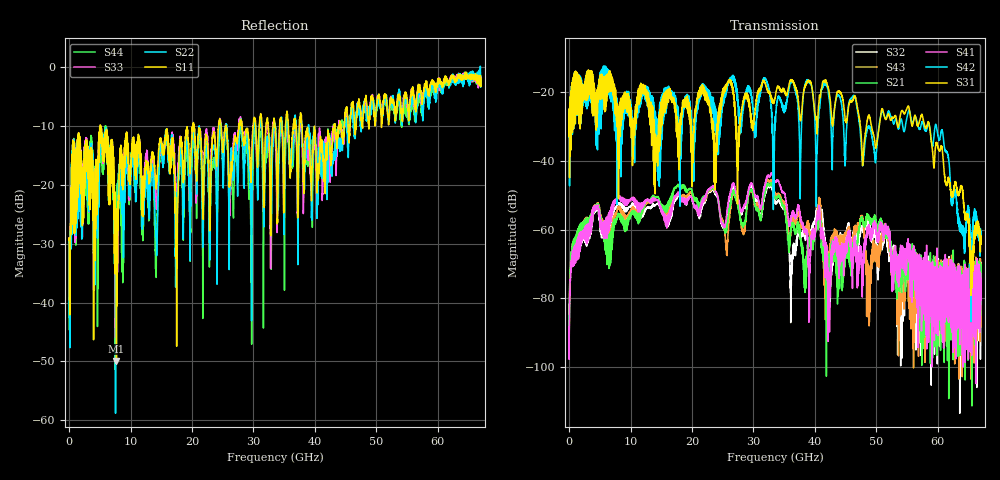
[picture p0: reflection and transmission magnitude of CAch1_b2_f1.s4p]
!Agilent Technologies,N5247A,US51170199,A.09.90.13
!Agilent N5247A: A.09.90.13
!Date: Thursday, October 18, 2018 12:09:48
!Correction: S11(Full 4 Port(1,2,3,4))
!S12(Full 4 Port(1,2,3,4))
!S13(Full 4 Port(1,2,3,4))
!S14(Full 4 Port(1,2,3,4))
!S21(Full 4 Port(1,2,3,4))
!S22(Full 4 Port(1,2,3,4))
!S23(Full 4 Port(1,2,3,4))
!S24(Full 4 Port(1,2,3,4))
!S31(Full 4 Port(1,2,3,4))
!S32(Full 4 Port(1,2,3,4))
!S33(Full 4 Port(1,2,3,4))
!S34(Full 4 Port(1,2,3,4))
!S41(Full 4 Port(1,2,3,4))
!S42(Full 4 Port(1,2,3,4))
!S43(Full 4 Port(1,2,3,4))
!S44(Full 4 Port(1,2,3,4))
!S4P File: Measurements: <S11,S12,S13,S14>,
!<S21,S22,S23,S24>,
!<S31,S32,S33,S34>,
!<S41,S42,S43,S44>:
# Hz S  dB  R 50
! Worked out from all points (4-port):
!   6701 points, 10 MHz to 67 GHz, reference 50 ohm
!   strongest paths, dB at 10 MHz, 16.76 GHz, 33.51 GHz, 50.25 GHz, 67 GHz:
!     S31: -32.9, -22.8, -21.9, -32.7, -63.0
!     S42: -33.1, -20.0, -29.9, -32.3, -62.8
!     S41: -88.2, -54.2, -46.0, -61.6, -80.5
!     S21: -87.9, -50.6, -50.5, -60.2, -77.4
!     S43: -87.8, -53.1, -49.3, -66.8, -77.2
!     S32: -81.7, -55.0, -52.3, -68.5, -69.5
!   lowest |S11| = -49.9 dB at 7.709 GHz (marker M1), VSWR 1.01, Z = 50.3 - j0.136 ohm
!   |S11| at or under -10 dB: start of sweep to 5.072 GHz; 5.182 GHz to 20.11 GHz (14.93 GHz wide, 118 % of centre); 37.91 GHz to 43.08 GHz (5.174 GHz wide, 12.8 % of centre)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
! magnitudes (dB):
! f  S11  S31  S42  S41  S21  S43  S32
! 10 MHz  -29.3  -32.9  -33.1  -88.2  -87.9  -87.8  -81.7
! 5.879 GHz  -11.5  -15.5  -12.6  -62.6  -63.9  -63.1  -63.7
! 7.709 GHz  -49.9  -26.9  -33.8  -51.2  -57.0  -54.9  -53.2
! 32.58 GHz  -12.9  -20.3  -20.2  -44.7  -47.1  -45.9  -47.4
! 42.24 GHz  -12.1  -19.3  -21.1  -79.8  -79.6  -70.4  -71.8
! 55.11 GHz  -6.6  -24.2  -26.4  -65.5  -69.5  -68.5  -73.3
! 67 GHz  -3.2  -63.0  -62.8  -80.5  -77.4  -77.2  -69.5
